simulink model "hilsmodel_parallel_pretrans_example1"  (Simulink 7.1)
settings: Solver=ode3  SolverMode=SingleTasking  StartTime=0.0  StopTime=1800  FixedStep=hilsmdl.simulation.stepsize.value  MaxStep=0.01  RelTol=1e-3  AbsTol=1e-3
undefined symbols (not defined in the file or in its folder): hilsmdl
libraries: HILS_model_library x10, simulink_extras x1, simulink x1

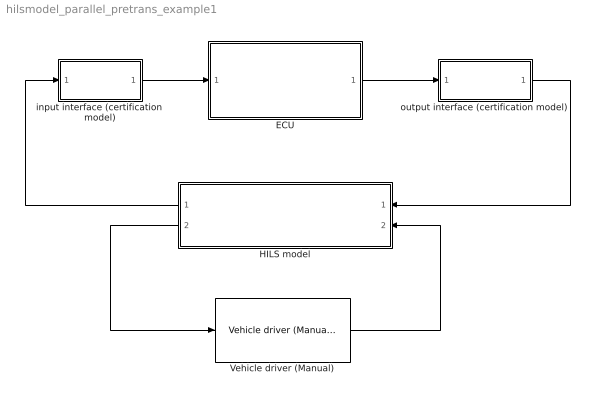
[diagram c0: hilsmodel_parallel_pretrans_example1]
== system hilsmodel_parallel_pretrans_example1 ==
  ECU : Subsystem  mask{dat=hilsmdl.ecu}
      mask prompts: dat "Data set for ECU"
  HILS model : Subsystem  Orientation=left
  Vehicle driver (Manual) : HILS_model_library/Driver/Vehicle driver (Manual)  dat=hilsmdl.drivermanual
  input interface (certification model) : Subsystem
  output interface (certification model) : Subsystem
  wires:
  input interface (certification model)/1(to ECU) -> ECU/1(sensor in)
  ECU/1(cmd out) -> output interface (certification model)/1(from ECU)
  HILS model/1(To Ctrl) -> input interface (certification model)/1(plant in)
  output interface (certification model)/1(cmd out) -> HILS model/1(From Ctrl)
  Vehicle driver (Manual)/1 -> HILS model/2(From Driver)
  HILS model/2(To driver) -> Vehicle driver (Manual)/1

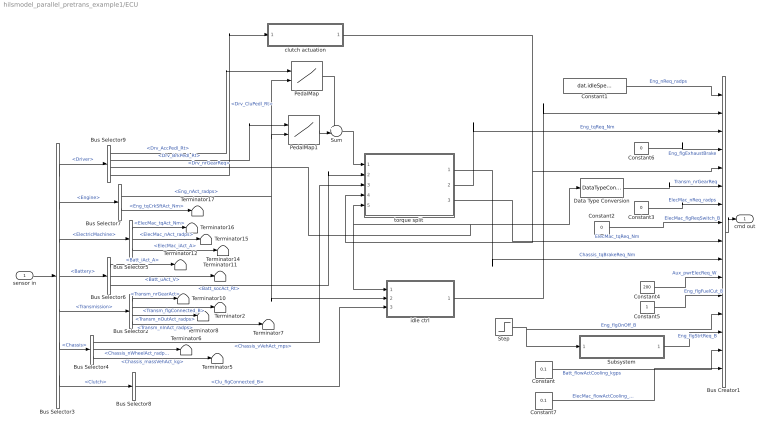
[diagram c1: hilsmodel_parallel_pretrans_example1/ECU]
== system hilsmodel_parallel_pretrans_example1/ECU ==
  sensor in : Inport
  Bus Creator1 : BusCreator  Inputs=16
  Bus Selector2 : BusSelector  OutputSignals=Transm_nrGearAct,Transm_flgConnected_B,Transm_nOutAct_radps,Transm_nInAct_radps
  Bus Selector3 : BusSelector  OutputSignals=Driver,Engine,ElectricMachine,Battery,Transmission,Chassis,Clutch
  Bus Selector4 : BusSelector  OutputSignals=Chassis_vVehAct_mps,Chassis_nWheelAct_radps,Chassis_massVehAct_kg
  Bus Selector5 : BusSelector  OutputSignals=ElecMac_tqAct_Nm,ElecMac_nAct_radps,ElecMac_iAct_A
  Bus Selector6 : BusSelector  OutputSignals=Batt_iAct_A,Batt_uAct_V,Batt_socAct_Rt
  Bus Selector7 : BusSelector  OutputSignals=Eng_nAct_radps,Eng_tqCrkSftAct_Nm
  Bus Selector8 : BusSelector  OutputSignals=Clu_flgConnected_B
  Bus Selector9 : BusSelector  OutputSignals=Drv_AccPedl_Rt,Drv_BrkPedl_Rt,Drv_nrGearReq,Drv_CluPedl_Rt
  Constant : Constant  Value=0.1
  Constant1 : Constant  Value=dat.idleSpeed.value
  Constant2 : Constant  Value=0
  Constant3 : Constant  Value=0
  Constant4 : Constant  Value=200
  Constant5 : Constant
  Constant6 : Constant  Value=0
  Constant7 : Constant  Value=0.1
  Data Type Conversion : DataTypeConversion
  PedalMap : Lookup2D  RowIndex=dat.pedalmap.pedal  ColumnIndex=dat.pedalmap.speed  Table=dat.pedalmap.map
  PedalMap1 : Lookup2D  RowIndex=dat.pedalmap.pedal  ColumnIndex=dat.pedalmap.speed  Table=2*dat.pedalmap.map
  Step : Step  SampleTime=0
  Subsystem : Subsystem
  Sum : Sum  Inputs=+-|
  Terminator{2,5..8,10..12,14..17} (12 alike) : Terminator
  clutch actuation : Subsystem
  idle ctrl : Subsystem
  torque split : Subsystem
  cmd out : Outport
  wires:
  Bus Selector3/6 -> Bus Selector4/1  "<Chassis>"
  Bus Selector3/5 -> Bus Selector2/1  "<Transmission>"
  Bus Selector3/3 -> Bus Selector5/1  "<ElectricMachine>"
  Bus Selector3/4 -> Bus Selector6/1  "<Battery>"
  sensor in/1 -> Bus Selector3/1
  Bus Creator1/1 -> cmd out/1
  Bus Selector6/1 -> Terminator12/1  "<Batt_iAct_A>"
  Bus Selector6/2 -> Terminator11/1  "<Batt_uAct_V>"
  Bus Selector6/3 -> torque split/2(SOC [0_1])  "<Batt_socAct_Rt>"
  Bus Selector2/1 -> Terminator10/1  "<Transm_nrGearAct>"
  Bus Selector2/2 -> Terminator2/1  "<Transm_flgConnected_B>"
  Bus Selector2/3 -> Terminator8/1  "<Transm_nOutAct_radps>"
  Bus Selector2/4 -> Terminator7/1  "<Transm_nInAct_radps>"
  Bus Selector5/3 -> Terminator14/1  "<ElecMac_iAct_A>"
  Bus Selector5/2 -> Terminator15/1  "<ElecMac_nAct_radps>"
  Bus Selector5/1 -> Terminator16/1  "<ElecMac_tqAct_Nm>"
  Bus Selector3/2 -> Bus Selector7/1  "<Engine>"
  Bus Selector7/2 -> Terminator17/1  "<Eng_tqCrkSftAct_Nm>"
  Bus Selector7/1 -> PedalMap/2, PedalMap1/2, idle ctrl/2(ICE_speed)  "<Eng_nAct_radps>"
  Bus Selector4/1 -> torque split/3(vehicle speed [m/s])  "<Chassis_vVehAct_mps>"
  Bus Selector4/2 -> Terminator6/1  "<Chassis_nWheelAct_radps>"
  Bus Selector4/3 -> Terminator5/1  "<Chassis_massVehAct_kg>"
  Bus Selector8/1 -> idle ctrl/3(CL_flag)  "<Clu_flgConnected_B>"
  PedalMap1/1 -> Sum/2
  PedalMap/1 -> Sum/1
  Sum/1 -> torque split/1(Tdemand [Nm])
  Bus Selector3/1 -> Bus Selector9/1  "<Driver>"
  Bus Selector9/1 -> PedalMap/1  "<Drv_AccPedl_Rt>"
  Bus Selector9/2 -> PedalMap1/1  "<Drv_BrkPedl_Rt>"
  Bus Selector3/7 -> Bus Selector8/1  "<Clutch>"
  Constant2/1 -> Bus Creator1/8  "ElecMac_flgReqSwitch_B"
  Constant3/1 -> Bus Creator1/7  "ElecMac_nReq_radps"
  Constant1/1 -> Bus Creator1/1  "Eng_nReq_radps"
  torque split/2(Treqice) -> Bus Creator1/3  "Eng_tqReq_Nm"
  torque split/3(Treqem) -> Bus Creator1/9  "ElecMac_tqReq_Nm"
  Constant6/1 -> Bus Creator1/4  "Eng_flgExhaustBrake"
  torque split/1(Tbrake) -> Bus Creator1/10  "Chassis_tqBrakeReq_Nm"
  Constant4/1 -> Bus Creator1/11  "Aux_pwrElecReq_W"
  Bus Selector9/3 -> Data Type Conversion/1, idle ctrl/1(gear), torque split/5(Gear [0_5])  "<Drv_nrGearReq>"
  Data Type Conversion/1 -> Bus Creator1/6  "Transm_nrGearReq"
  Bus Selector9/4 -> clutch actuation/1(In1)  "<Drv_CluPedl_Rt>"
  clutch actuation/1(Out1) -> torque split/4(Clutch [0;1]), Bus Creator1/5
  idle ctrl/1(Out1) -> Bus Creator1/2
  Constant5/1 -> Bus Creator1/12  "Eng_flgFuelCut_B"
  Step/1 -> Subsystem/1(Engine onoff), Bus Creator1/13  "Eng_flgOnOff_B"
  Subsystem/1(Starter motor ctrl) -> Bus Creator1/14  "Eng_flgStrtReq_B"
  Constant/1 -> Bus Creator1/15  "Batt_flowActCooling_kgps"
  Constant7/1 -> Bus Creator1/16  "ElecMac_flowActCooling_kgps"

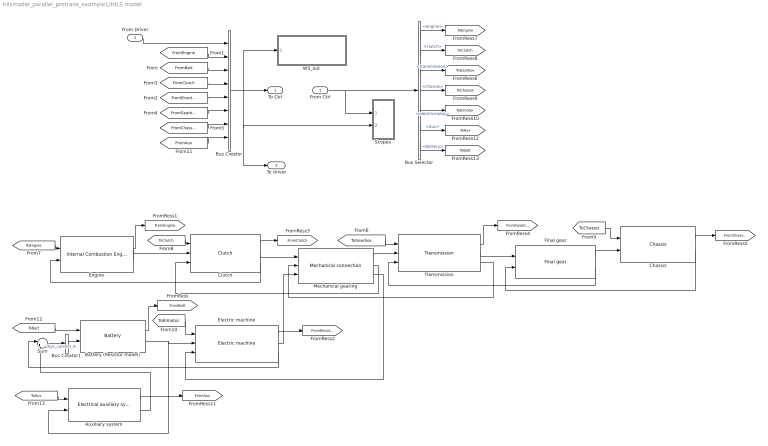
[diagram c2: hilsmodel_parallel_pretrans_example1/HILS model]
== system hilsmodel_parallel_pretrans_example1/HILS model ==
  From Ctrl : Inport
  From Driver : Inport  Port=2
  Auxiliary system : HILS_model_library/Auxiliary systems/Electrical auxiliary system
  Battery (Resistor model) : HILS_model_library/Rechargable energy storage systems/Battery  dat=hilsmdl.battery
  Bus Creator : BusCreator  Inputs=8
  Bus Creator1 : BusCreator  Inputs=1
  Bus Selector : BusSelector  OutputSignals=engine,clutch,transmission,chassis,electricmotor,aux,Battery
  Chassis : HILS_model_library/Chassis/Chassis  dat=hilsmdl.chassis
  Clutch : HILS_model_library/Mechanical components/Clutch  dat=hilsmdl.clutch
  Electric machine : HILS_model_library/Energy converters/Electric machine  dat=hilsmdl.elmachine
  Engine : HILS_model_library/Energy converters/Internal Combustion Engine  dat=hilsmdl.eng
  Final gear : HILS_model_library/Mechanical components/Final gear  dat=hilsmdl.finalgear
  Mechanical gearing : HILS_model_library/Mechanical components/Mechanical connection  dat=hilsmdl.mechconnection
  Scopes : Subsystem
  Sum : Sum  Inputs=|++
  Transmission : HILS_model_library/Mechanical components/Transmission  dat=hilsmdl.transmission
  WS_out : Subsystem
  To Ctrl : Outport
  To driver : Outport  Port=2
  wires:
  From Driver/1 -> Bus Creator/1
  Battery (Resistor model)/2 -> Electric machine/2, Auxiliary system/2
  Mechanical gearing/3 -> Electric machine/3
  Mechanical gearing/1 -> Transmission/2
  Bus Creator/1 -> To Ctrl/1, To driver/1, Scopes/2(plnt in), WS_out/1(from model)
  Clutch/2 -> Mechanical gearing/1
  Mechanical gearing/2 -> Clutch/3
  Clutch/3 -> Engine/2
  Transmission/3 -> Mechanical gearing/2
  Engine/2 -> Clutch/2
  Chassis/1 -> [FromChassis]
  From Ctrl/1 -> Scopes/1(ctrl in), Bus Selector/1
  Electric machine/2 -> Mechanical gearing/3
  Battery (Resistor model)/1 -> [FromBatt]
  [FromBatt] -> Bus Creator/3
  Engine/1 -> [FromEngine]
  [FromEngine] -> Bus Creator/2
  [FromElmotor] -> Bus Creator/5
  Electric machine/1 -> [FromElmotor]
  [FromClutch] -> Bus Creator/4
  Clutch/1 -> [FromClutch]
  [FromGearbox] -> Bus Creator/6
  Transmission/1 -> [FromGearbox]
  [FromChassis] -> Bus Creator/7
  Bus Selector/3 -> [ToGearbox]  "<transmission>"
  [ToGearbox] -> Transmission/1
  Bus Selector/1 -> [ToEngine]  "<engine>"
  Bus Selector/2 -> [ToClutch]  "<clutch>"
  Bus Selector/4 -> [ToChassis]  "<chassis>"
  Bus Selector/5 -> [ToElmotor]  "<electricmotor>"
  [ToEngine] -> Engine/1
  [ToClutch] -> Clutch/1
  [ToChassis] -> Chassis/1
  [ToElmotor] -> Electric machine/1
  [ToBatt] -> Battery (Resistor model)/1
  [ToAux] -> Auxiliary system/1
  Auxiliary system/1 -> [FromAux]
  [FromAux] -> Bus Creator/8
  Auxiliary system/2 -> Sum/2
  Electric machine/3 -> Sum/1
  Bus Creator1/1 -> Battery (Resistor model)/2
  Sum/1 -> Bus Creator1/1  "phys_current_A"
  Bus Selector/6 -> [ToAux]  "<aux>"
  Transmission/2 -> Final gear/1
  Final gear/2 -> Transmission/3
  Final gear/1 -> Chassis/2
  Chassis/2 -> Final gear/2
  Bus Selector/7 -> [ToBatt]  "<Battery>"

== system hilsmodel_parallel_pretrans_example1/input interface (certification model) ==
  plant in : Inport
  Bus Creator : BusCreator  Inputs=35
  Bus Selector : BusSelector  OutputSignals=Driver,Driver.Drv_AccPedl_Rt,Driver.Drv_BrkPedl_Rt,Driver.Drivecycle_RefSpeed_mps,Driver.Drv_CluPedl_Rt,Driver.Drv_nrGearReq,Engine,Engine.Eng_nAct_radps,Engine.Eng_tqCrkSftAct_Nm,Engine.Eng_tqIndAct_Nm,Engine.Eng_tOilAct_K,Battery,Battery.Batt_iAct_A,Battery.Batt_uAct_V,Battery.Batt_socAct_Rt,Battery.Batt_tAct_K,Clutch,Clutch.Clu_flgConnected_B,ElectricMachine,ElectricMachine.ElecMac_tqAct_Nm,Ele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
  to ECU : Outport
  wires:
  plant in/1 -> Bus Selector/1
  Bus Selector/1 -> Bus Creator/1  "<Driver>"
  Bus Selector/2 -> Bus Creator/2  "<Drv_AccPedl_Rt>"
  Bus Selector/3 -> Bus Creator/3  "<Drv_BrkPedl_Rt>"
  Bus Selector/4 -> Bus Creator/4  "<Drivecycle_RefSpeed_mps>"
  Bus Selector/5 -> Bus Creator/5  "<Drv_CluPedl_Rt>"
  Bus Selector/7 -> Bus Creator/7  "<Engine>"
  Bus Selector/8 -> Bus Creator/8  "<Eng_nAct_radps>"
  Bus Selector/9 -> Bus Creator/9  "<Eng_tqCrkSftAct_Nm>"
  Bus Selector/6 -> Bus Creator/6  "<Drv_nrGearReq>"
  Bus Creator/1 -> to ECU/1
  Bus Selector/10 -> Bus Creator/10  "<Eng_tqIndAct_Nm>"
  Bus Selector/11 -> Bus Creator/11  "<Eng_tOilAct_K>"
  Bus Selector/12 -> Bus Creator/12  "<Battery>"
  Bus Selector/13 -> Bus Creator/13  "<Batt_iAct_A>"
  Bus Selector/14 -> Bus Creator/14  "<Batt_uAct_V>"
  Bus Selector/15 -> Bus Creator/15  "<Batt_socAct_Rt>"
  Bus Selector/16 -> Bus Creator/16  "<Batt_tAct_K>"
  Bus Selector/17 -> Bus Creator/17  "<Clutch>"
  Bus Selector/18 -> Bus Creator/18  "<Clu_flgConnected_B>"
  Bus Selector/19 -> Bus Creator/19  "<ElectricMachine>"
  Bus Selector/20 -> Bus Creator/20  "<ElecMac_tqAct_Nm>"
  Bus Selector/21 -> Bus Creator/21  "<ElecMac_nAct_radps>"
  Bus Selector/22 -> Bus Creator/22  "<ElecMac_iAct_A>"
  Bus Selector/23 -> Bus Creator/23  "<ElecMac_tAct_K>"
  Bus Selector/24 -> Bus Creator/24  "<Transmission>"
  Bus Selector/25 -> Bus Creator/25  "<Transm_nOutAct_radps>"
  Bus Selector/26 -> Bus Creator/26  "<Transm_nrGearAct>"
  Bus Selector/27 -> Bus Creator/27  "<Transm_flgConnected_B>"
  Bus Selector/28 -> Bus Creator/28  "<Transm_nInAct_radps>"
  Bus Selector/29 -> Bus Creator/29  "<Chassis>"
  Bus Selector/30 -> Bus Creator/30  "<Chassis_vVehAct_mps>"
  Bus Selector/31 -> Bus Creator/31  "<Chassis_nWheelAct_radps>"
  Bus Selector/32 -> Bus Creator/32  "<Chassis_massVehAct_kg>"
  Bus Selector/33 -> Bus Creator/33  "<Chassis_slopRoad_rad>"
  Bus Selector/34 -> Bus Creator/34  "<Auxiliary>"
  Bus Selector/35 -> Bus Creator/35  "<Aux_iAct_A>"

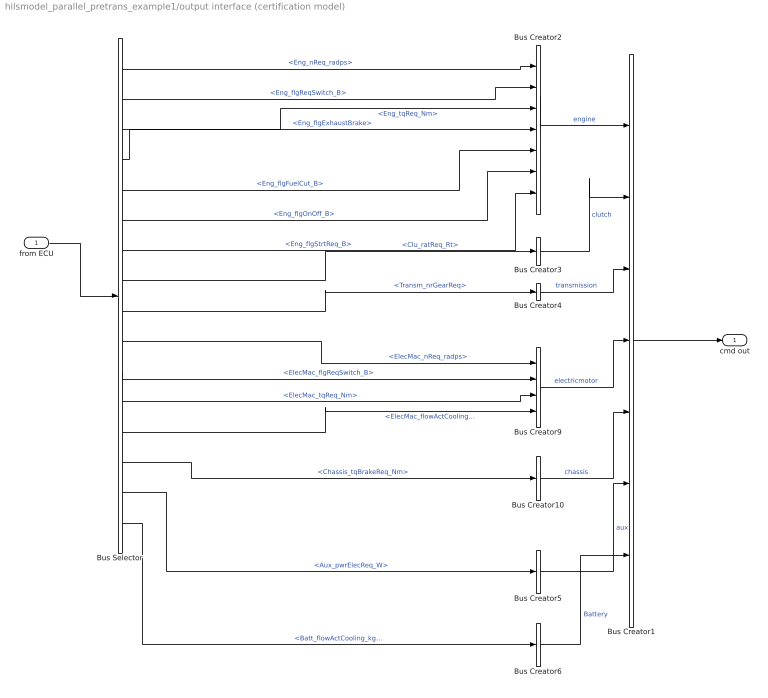
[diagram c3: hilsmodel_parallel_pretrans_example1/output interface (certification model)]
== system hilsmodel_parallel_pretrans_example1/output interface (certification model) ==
  from ECU : Inport
  Bus Creator1 : BusCreator  Inputs=7
  Bus Creator{3..6,10} (5 alike) : BusCreator  Inputs=1
  Bus Creator2 : BusCreator  Inputs=7
  Bus Creator9 : BusCreator
  Bus Selector : BusSelector  OutputSignals=Eng_nReq_radps,Eng_flgReqSwitch_B,Eng_tqReq_Nm,Eng_flgExhaustBrake,Eng_flgFuelCut_B,Eng_flgOnOff_B,Eng_flgStrtReq_B,Clu_ratReq_Rt,Transm_nrGearReq,ElecMac_nReq_radps,ElecMac_flgReqSwitch_B,ElecMac_tqReq_Nm,ElecMac_flowActCooling_kgps,Chassis_tqBrakeReq_Nm,Aux_pwrElecReq_W,Batt_flowActCooling_kgps
  cmd out : Outport
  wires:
  from ECU/1 -> Bus Selector/1
  Bus Creator4/1 -> Bus Creator1/3  "transmission"
  Bus Creator3/1 -> Bus Creator1/2  "clutch"
  Bus Creator10/1 -> Bus Creator1/5  "chassis"
  Bus Creator9/1 -> Bus Creator1/4  "electricmotor"
  Bus Selector/11 -> Bus Creator9/2  "<ElecMac_flgReqSwitch_B>"
  Bus Selector/10 -> Bus Creator9/1  "<ElecMac_nReq_radps>"
  Bus Creator1/1 -> cmd out/1
  Bus Creator2/1 -> Bus Creator1/1  "engine"
  Bus Selector/1 -> Bus Creator2/1  "<Eng_nReq_radps>"
  Bus Selector/2 -> Bus Creator2/2  "<Eng_flgReqSwitch_B>"
  Bus Selector/3 -> Bus Creator2/3  "<Eng_tqReq_Nm>"
  Bus Selector/12 -> Bus Creator9/3  "<ElecMac_tqReq_Nm>"
  Bus Selector/4 -> Bus Creator2/4  "<Eng_flgExhaustBrake>"
  Bus Selector/8 -> Bus Creator3/1  "<Clu_ratReq_Rt>"
  Bus Selector/9 -> Bus Creator4/1  "<Transm_nrGearReq>"
  Bus Selector/14 -> Bus Creator10/1  "<Chassis_tqBrakeReq_Nm>"
  Bus Creator5/1 -> Bus Creator1/6  "aux"
  Bus Selector/15 -> Bus Creator5/1  "<Aux_pwrElecReq_W>"
  Bus Selector/5 -> Bus Creator2/5  "<Eng_flgFuelCut_B>"
  Bus Selector/6 -> Bus Creator2/6  "<Eng_flgOnOff_B>"
  Bus Selector/7 -> Bus Creator2/7  "<Eng_flgStrtReq_B>"
  Bus Selector/16 -> Bus Creator6/1  "<Batt_flowActCooling_kgps>"
  Bus Creator6/1 -> Bus Creator1/7  "Battery"
  Bus Selector/13 -> Bus Creator9/4  "<ElecMac_flowActCooling_kgps>"

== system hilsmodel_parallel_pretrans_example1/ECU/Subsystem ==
  Engine onoff : Inport
  Data Type Conversion : DataTypeConversion
  Data Type Conversion1 : DataTypeConversion
  S-R Flip-Flop : simulink_extras/Flip Flops/S-R Flip-Flop  initial_condition=0
  Terminator : Terminator
  Transport Delay : TransportDelay
  Starter motor ctrl : Outport
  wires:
  Engine onoff/1 -> Transport Delay/1, Data Type Conversion/1
  S-R Flip-Flop/1 -> Starter motor ctrl/1
  S-R Flip-Flop/2 -> Terminator/1
  Transport Delay/1 -> Data Type Conversion1/1
  Data Type Conversion/1 -> S-R Flip-Flop/1
  Data Type Conversion1/1 -> S-R Flip-Flop/2

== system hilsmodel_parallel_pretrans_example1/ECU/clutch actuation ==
  In1 : Inport
  Gain : Gain
  Scope : Scope
  Out1 : Outport
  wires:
  In1/1 -> Gain/1
  Gain/1 -> Out1/1, Scope/1  "Clu_ratReq_Rt"

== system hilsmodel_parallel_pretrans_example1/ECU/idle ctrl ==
  gear : Inport
  ICE_speed : Inport  Port=2
  CL_flag : Inport  Port=3
  Compare To Zero : simulink/Logic and Bit Operations/Compare To Zero  relop=<=  LogicOutDataTypeMode=boolean
  Const2 : Constant  Value=dat.idleSpeed.value
  Logical Operator : Logic  Operator=NOT  AllPortsSameDT=off  OutDataTypeStr=boolean  OutDataTypeMode=boolean
  Logical Operator1 : Logic  Operator=OR  AllPortsSameDT=off  OutDataTypeStr=boolean  OutDataTypeMode=boolean
  Logical Operator2 : Logic  Operator=OR  AllPortsSameDT=off  OutDataTypeStr=boolean  OutDataTypeMode=boolean
  Relational Operator1 : RelationalOperator  Operator=<  OutDataTypeStr=boolean  LogicOutDataTypeMode=boolean
  Out1 : Outport
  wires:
  Compare To Zero/1 -> Logical Operator1/1
  Relational Operator1/1 -> Logical Operator2/1
  Const2/1 -> Relational Operator1/2
  gear/1 -> Compare To Zero/1
  ICE_speed/1 -> Relational Operator1/1
  Logical Operator1/1 -> Out1/1  "Eng_flgReqSwitch_B"
  Logical Operator2/1 -> Logical Operator1/2
  CL_flag/1 -> Logical Operator/1
  Logical Operator/1 -> Logical Operator2/2

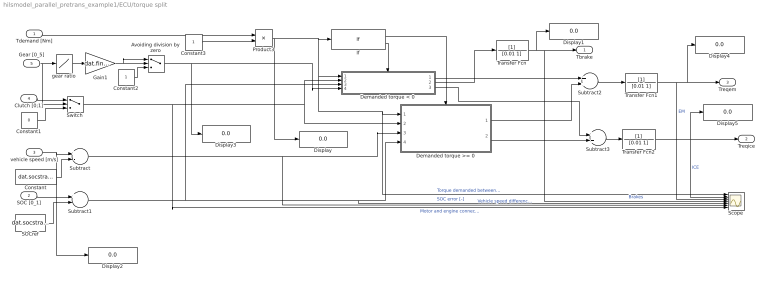
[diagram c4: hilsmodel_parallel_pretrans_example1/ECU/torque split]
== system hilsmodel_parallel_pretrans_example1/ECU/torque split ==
  Tdemand [Nm] : Inport
  SOC [0_1] : Inport  Port=2
  vehicle speed [m/s] : Inport  Port=3
  Clutch [0;1] : Inport  Port=4
  Gear [0_5] : Inport  Port=5
  Avoiding division by zero : Switch  Criteria=u2 > Threshold  Threshold=0.1
  Constant : Constant  Value=dat.socstrategy.SwitchSpeed
  Constant1 : Constant  Value=0
  Constant2 : Constant
  Constant3 : Constant
  Demanded torque < 0 : Subsystem  TreatAsAtomicUnit=on
  Demanded torque >= 0 : Subsystem  TreatAsAtomicUnit=on
  Display{,1..5} (6 alike) : Display
  Gain1 : Gain  Gain=dat.finalgear.value
  If : If  IfExpression=u1 >=0
  Product3 : Product  Inputs=*/
  SOCref : Constant  Value=dat.socstrategy.socref
  Scope : Scope  NumInputPorts=7
  Subtract : Sum  Inputs=+-
  Subtract1 : Sum  Inputs=+-
  Subtract2 : Sum
  Subtract3 : Sum
  Switch : Switch  Threshold=0.5
  Transfer Fcn : TransferFcn  Denominator=[0.01 1]
  Transfer Fcn1 : TransferFcn  Denominator=[0.01 1]
  Transfer Fcn2 : TransferFcn  Denominator=[0.01 1]
  gear ratio : Lookup  InputValues=dat.gearname.value  Table=dat.gearratio.value
  Tbrake : Outport
  Treqice : Outport  Port=2
  Treqem : Outport  Port=3
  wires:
  Gear [0_5]/1 -> gear ratio/1, Switch/2
  Tdemand [Nm]/1 -> Product3/1
  gear ratio/1 -> Gain1/1
  Product3/1 -> If/1, Demanded torque < 0/1(Tdemand [Nm]), Demanded torque >= 0/1(Tdemand [Nm]), Scope/1, Display/1  "Torque demanded between clutch and EM/ICE"
  Clutch [0;1]/1 -> Switch/1
  Constant1/1 -> Switch/3
  Switch/1 -> Demanded torque < 0/2(Connected? [0;1]), Demanded torque >= 0/2(Connected? [0;1]), Scope/7  "Motor and engine connected to wheels ?"
  vehicle speed [m/s]/1 -> Subtract/1, Display2/1
  Constant/1 -> Subtract/2
  Subtract/1 -> Demanded torque >= 0/3(Switch diff [m/s]), Scope/6  "Vehicle speed difference from  EM/ICE switch speed [m/s]"
  SOC [0_1]/1 -> Subtract1/1
  SOCref/1 -> Subtract1/2
  Subtract1/1 -> Demanded torque < 0/3(SOC error), Demanded torque >= 0/4(SOC error [-]), Scope/5  "SOC error [-]"
  If/1 -> Demanded torque >= 0/Action
  If/2 -> Demanded torque < 0/Action
  Demanded torque < 0/1(Torque EM) -> Subtract2/1
  Demanded torque >= 0/1(Torque EM) -> Subtract2/2
  Subtract2/1 -> Transfer Fcn1/1
  Demanded torque < 0/2(Torque brakes) -> Transfer Fcn/1
  Gain1/1 -> Avoiding division by zero/2, Avoiding division by zero/1
  Constant2/1 -> Avoiding division by zero/3
  Avoiding division by zero/1 -> Demanded torque < 0/4(Gear ratio), Display3/1
  Demanded torque >= 0/2(Torque ICE) -> Subtract3/2
  Demanded torque < 0/3(Torque ICE) -> Subtract3/1
  Subtract3/1 -> Transfer Fcn2/1
  Transfer Fcn/1 -> Display1/1, Tbrake/1, Scope/4  "Brakes"
  Transfer Fcn1/1 -> Treqem/1, Display4/1, Scope/3  "EM"
  Transfer Fcn2/1 -> Treqice/1, Display5/1, Scope/2  "ICE"
  Constant3/1 -> Product3/2

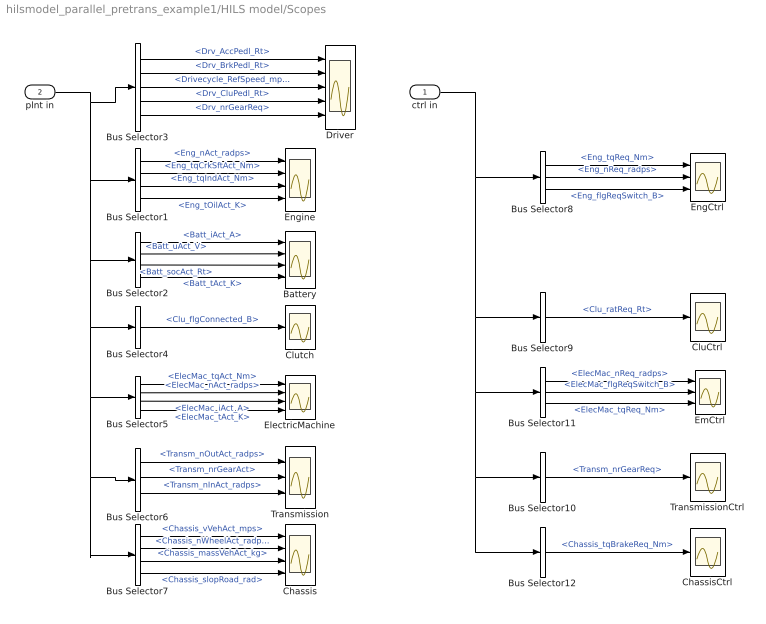
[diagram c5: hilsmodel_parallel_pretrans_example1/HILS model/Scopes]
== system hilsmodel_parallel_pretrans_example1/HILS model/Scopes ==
  ctrl in : Inport
  plnt in : Inport  Port=2
  Battery : Scope  NumInputPorts=4
  Bus Selector1 : BusSelector  OutputSignals=Engine.Eng_nAct_radps,Engine.Eng_tqCrkSftAct_Nm,Engine.Eng_tqIndAct_Nm,Engine.Eng_tOilAct_K
  Bus Selector10 : BusSelector  OutputSignals=transmission.Transm_nrGearReq
  Bus Selector11 : BusSelector  OutputSignals=electricmotor.ElecMac_nReq_radps,electricmotor.ElecMac_flgReqSwitch_B,electricmotor.ElecMac_tqReq_Nm
  Bus Selector12 : BusSelector  OutputSignals=chassis.Chassis_tqBrakeReq_Nm
  Bus Selector2 : BusSelector  OutputSignals=Battery.Batt_iAct_A,Battery.Batt_uAct_V,Battery.Batt_socAct_Rt,Battery.Batt_tAct_K
  Bus Selector3 : BusSelector  OutputSignals=Driver.Drv_AccPedl_Rt,Driver.Drv_BrkPedl_Rt,Driver.Drivecycle_RefSpeed_mps,Driver.Drv_CluPedl_Rt,Driver.Drv_nrGearReq
  Bus Selector4 : BusSelector  OutputSignals=Clutch.Clu_flgConnected_B
  Bus Selector5 : BusSelector  OutputSignals=ElectricMachine.ElecMac_tqAct_Nm,ElectricMachine.ElecMac_nAct_radps,ElectricMachine.ElecMac_iAct_A,ElectricMachine.ElecMac_tAct_K
  Bus Selector6 : BusSelector  OutputSignals=Transmission.Transm_nOutAct_radps,Transmission.Transm_nrGearAct,Transmission.Transm_nInAct_radps,Transmission.Transm_flgConnected_B
  Bus Selector7 : BusSelector  OutputSignals=Chassis.Chassis_vVehAct_mps,Chassis.Chassis_nWheelAct_radps,Chassis.Chassis_massVehAct_kg,Chassis.Chassis_slopRoad_rad
  Bus Selector8 : BusSelector  OutputSignals=engine.Eng_tqReq_Nm,engine.Eng_nReq_radps,engine.Eng_flgReqSwitch_B
  Bus Selector9 : BusSelector  OutputSignals=clutch.Clu_ratReq_Rt
  Chassis : Scope  NumInputPorts=4
  ChassisCtrl : Scope
  CluCtrl : Scope
  Clutch : Scope
  Driver : Scope  NumInputPorts=5
  ElectricMachine : Scope  NumInputPorts=4
  EmCtrl : Scope  NumInputPorts=3
  EngCtrl : Scope  NumInputPorts=3
  Engine : Scope  NumInputPorts=4
  Transmission : Scope  NumInputPorts=3
  TransmissionCtrl : Scope
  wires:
  Bus Selector3/1 -> Driver/1  "<Drv_AccPedl_Rt>"
  Bus Selector3/3 -> Driver/3  "<Drivecycle_RefSpeed_mps>"
  Bus Selector3/2 -> Driver/2  "<Drv_BrkPedl_Rt>"
  plnt in/1 -> Bus Selector3/1, Bus Selector1/1, Bus Selector2/1, Bus Selector4/1, Bus Selector5/1, Bus Selector6/1, Bus Selector7/1
  Bus Selector1/1 -> Engine/1  "<Eng_nAct_radps>"
  Bus Selector1/2 -> Engine/2  "<Eng_tqCrkSftAct_Nm>"
  Bus Selector2/1 -> Battery/1  "<Batt_iAct_A>"
  Bus Selector2/2 -> Battery/2  "<Batt_uAct_V>"
  Bus Selector2/3 -> Battery/3  "<Batt_socAct_Rt>"
  Bus Selector4/1 -> Clutch/1  "<Clu_flgConnected_B>"
  Bus Selector5/1 -> ElectricMachine/1  "<ElecMac_tqAct_Nm>"
  Bus Selector5/2 -> ElectricMachine/2  "<ElecMac_nAct_radps>"
  Bus Selector6/1 -> Transmission/1  "<Transm_nOutAct_radps>"
  Bus Selector6/2 -> Transmission/2  "<Transm_nrGearAct>"
  Bus Selector6/3 -> Transmission/3  "<Transm_nInAct_radps>"
  Bus Selector7/1 -> Chassis/1  "<Chassis_vVehAct_mps>"
  Bus Selector7/2 -> Chassis/2  "<Chassis_nWheelAct_radps>"
  Bus Selector7/3 -> Chassis/3  "<Chassis_massVehAct_kg>"
  Bus Selector7/4 -> Chassis/4  "<Chassis_slopRoad_rad>"
  ctrl in/1 -> Bus Selector8/1, Bus Selector9/1, Bus Selector11/1, Bus Selector10/1, Bus Selector12/1
  Bus Selector8/1 -> EngCtrl/1  "<Eng_tqReq_Nm>"
  Bus Selector8/2 -> EngCtrl/2  "<Eng_nReq_radps>"
  Bus Selector9/1 -> CluCtrl/1  "<Clu_ratReq_Rt>"
  Bus Selector10/1 -> TransmissionCtrl/1  "<Transm_nrGearReq>"
  Bus Selector11/1 -> EmCtrl/1  "<ElecMac_nReq_radps>"
  Bus Selector11/2 -> EmCtrl/2  "<ElecMac_flgReqSwitch_B>"
  Bus Selector11/3 -> EmCtrl/3  "<ElecMac_tqReq_Nm>"
  Bus Selector12/1 -> ChassisCtrl/1  "<Chassis_tqBrakeReq_Nm>"
  Bus Selector8/3 -> EngCtrl/3  "<Eng_flgReqSwitch_B>"
  Bus Selector1/3 -> Engine/3  "<Eng_tqIndAct_Nm>"
  Bus Selector1/4 -> Engine/4  "<Eng_tOilAct_K>"
  Bus Selector2/4 -> Battery/4  "<Batt_tAct_K>"
  Bus Selector5/3 -> ElectricMachine/3  "<ElecMac_iAct_A>"
  Bus Selector5/4 -> ElectricMachine/4  "<ElecMac_tAct_K>"
  Bus Selector3/4 -> Driver/4  "<Drv_CluPedl_Rt>"
  Bus Selector3/5 -> Driver/5  "<Drv_nrGearReq>"

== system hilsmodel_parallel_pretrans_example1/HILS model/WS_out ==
  from model : Inport
  To Workspace : ToWorkspace  VariableName=certmdl_out  SampleTime=hilsmdl.simulation.sampletime.value  SaveFormat=Structure With Time
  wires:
  from model/1 -> To Workspace/1

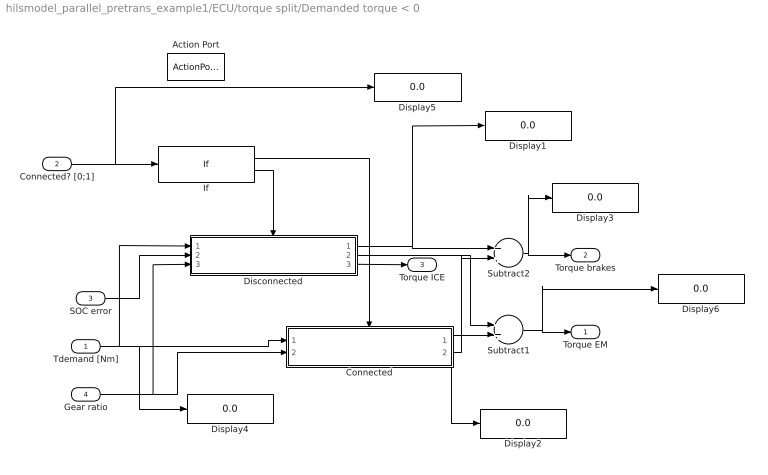
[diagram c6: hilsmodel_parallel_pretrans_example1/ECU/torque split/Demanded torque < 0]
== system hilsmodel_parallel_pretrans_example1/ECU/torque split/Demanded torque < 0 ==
  Tdemand [Nm] : Inport
  Connected? [0;1] : Inport  Port=2
  SOC error : Inport  Port=3
  Gear ratio : Inport  Port=4
  Action Port : ActionPort  InitializeStates=reset  ActionType=else
  Connected : Subsystem  TreatAsAtomicUnit=on
  Disconnected : Subsystem  TreatAsAtomicUnit=on
  Display{1..6} (6 alike) : Display
  If : If  IfExpression=u1 > 0.5
  Subtract1 : Sum
  Subtract2 : Sum
  Torque EM : Outport  OutputWhenDisabled=reset  InitialOutput=[0]
  Torque brakes : Outport  Port=2  OutputWhenDisabled=reset  InitialOutput=[0]
  Torque ICE : Outport  Port=3
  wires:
  If/1 -> Connected/Action
  If/2 -> Disconnected/Action
  Disconnected/1(Torque brakes) -> Subtract2/1, Display1/1
  Connected/2(Torque brakes) -> Subtract2/2, Display2/1
  Subtract2/1 -> Torque brakes/1, Display3/1
  Tdemand [Nm]/1 -> Disconnected/1(Tdemand [Nm]), Connected/1(Tdemand [Nm]), Display4/1
  Connected/1(Torque EM) -> Subtract1/2
  Disconnected/2(Torque EM) -> Subtract1/1
  Subtract1/1 -> Torque EM/1, Display6/1
  Disconnected/3(Torque ICE) -> Torque ICE/1
  SOC error/1 -> Disconnected/2(SOC error)
  Connected? [0;1]/1 -> If/1, Display5/1
  Gear ratio/1 -> Connected/2(Gear ratio), Disconnected/3(Gear ratio)

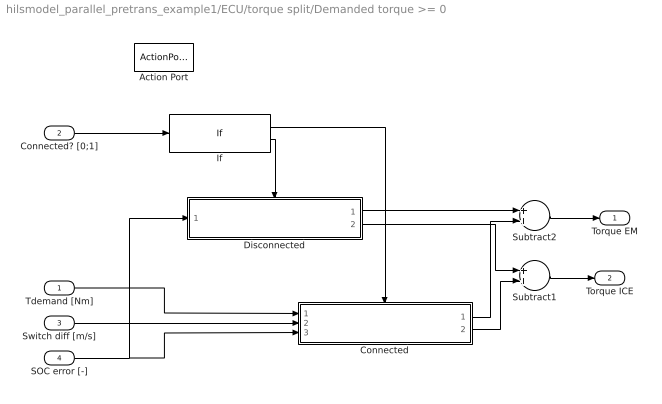
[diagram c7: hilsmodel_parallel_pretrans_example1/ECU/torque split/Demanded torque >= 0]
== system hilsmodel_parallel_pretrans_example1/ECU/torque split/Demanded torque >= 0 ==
  Tdemand [Nm] : Inport
  Connected? [0;1] : Inport  Port=2
  Switch diff [m/s] : Inport  Port=3
  SOC error [-] : Inport  Port=4
  Action Port : ActionPort  InitializeStates=reset  ActionType=then
  Connected : Subsystem  TreatAsAtomicUnit=on
  Disconnected : Subsystem  TreatAsAtomicUnit=on
  If : If  IfExpression=u1 > 0.5
  Subtract1 : Sum
  Subtract2 : Sum
  Torque EM : Outport  OutputWhenDisabled=reset  InitialOutput=[0]
  Torque ICE : Outport  Port=2  OutputWhenDisabled=reset  InitialOutput=[0]
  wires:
  If/1 -> Connected/Action
  If/2 -> Disconnected/Action
  Connected? [0;1]/1 -> If/1
  Switch diff [m/s]/1 -> Connected/2(Switch diff [m/s])
  SOC error [-]/1 -> Connected/3(SOC error), Disconnected/1(SOC error)
  Connected/1(Torque EM) -> Subtract2/2
  Tdemand [Nm]/1 -> Connected/1(Tdemand [Nm])
  Disconnected/1(Torque EM) -> Subtract2/1
  Connected/2(Torque ICE) -> Subtract1/2
  Disconnected/2(Torque ICE) -> Subtract1/1
  Subtract2/1 -> Torque EM/1
  Subtract1/1 -> Torque ICE/1

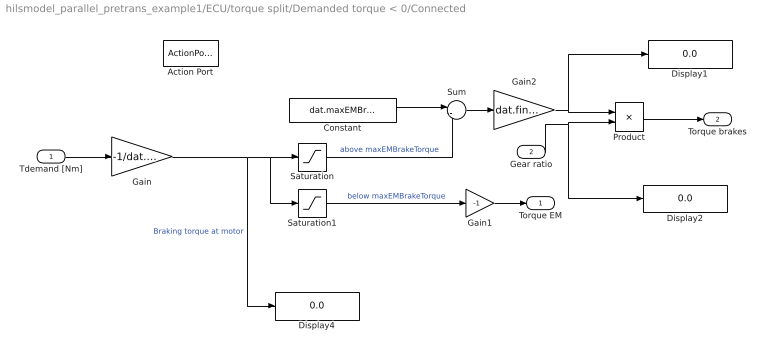
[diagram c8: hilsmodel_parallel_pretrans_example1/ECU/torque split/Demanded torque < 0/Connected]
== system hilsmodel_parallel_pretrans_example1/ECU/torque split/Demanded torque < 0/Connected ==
  Tdemand [Nm] : Inport
  Gear ratio : Inport  Port=2
  Action Port : ActionPort  InitializeStates=reset  ActionType=then
  Constant : Constant  Value=dat.maxEMBrakeTorque.value
  Display1 : Display
  Display2 : Display
  Display4 : Display
  Gain : Gain  Gain=-1/dat.finalgear.value
  Gain1 : Gain  Gain=-1
  Gain2 : Gain  Gain=dat.finalgear.value
  Product : Product
  Saturation : Saturate  UpperLimit=inf  LowerLimit=dat.maxEMBrakeTorque.value
  Saturation1 : Saturate  UpperLimit=dat.maxEMBrakeTorque.value  LowerLimit=-inf
  Sum : Sum  Inputs=|-+
  Torque EM : Outport  OutputWhenDisabled=reset  InitialOutput=[0]
  Torque brakes : Outport  Port=2  OutputWhenDisabled=reset  InitialOutput=[0]
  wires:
  Tdemand [Nm]/1 -> Gain/1
  Gain/1 -> Saturation/1, Saturation1/1, Display4/1  "Braking torque at motor"
  Saturation1/1 -> Gain1/1  "below maxEMBrakeTorque"
  Saturation/1 -> Sum/2  "above maxEMBrakeTorque"
  Constant/1 -> Sum/1
  Sum/1 -> Gain2/1
  Gain1/1 -> Torque EM/1
  Gain2/1 -> Display1/1, Product/1
  Product/1 -> Torque brakes/1
  Gear ratio/1 -> Product/2, Display2/1

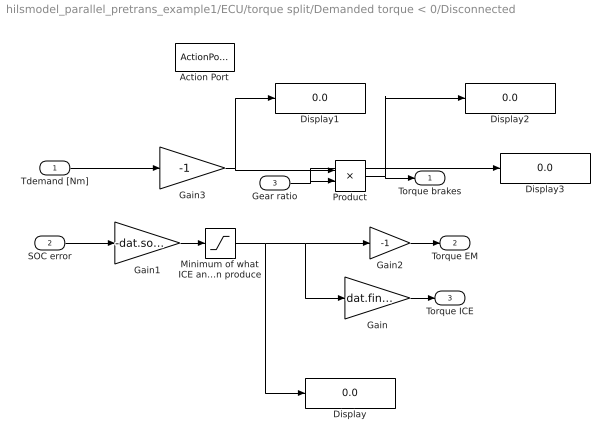
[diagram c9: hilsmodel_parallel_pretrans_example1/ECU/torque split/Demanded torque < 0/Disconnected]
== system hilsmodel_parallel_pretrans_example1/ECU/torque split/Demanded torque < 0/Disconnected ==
  Tdemand [Nm] : Inport
  SOC error : Inport  Port=2
  Gear ratio : Inport  Port=3
  Action Port : ActionPort  InitializeStates=reset  ActionType=else
  Display{,1..3} (4 alike) : Display
  Gain : Gain  Gain=dat.finalgear.value
  Gain1 : Gain  Gain=-dat.socstrategy.Ksoc
  Gain2 : Gain  Gain=-1
  Gain3 : Gain  Gain=-1
  Minimum of what ICE and EM can produce : Saturate  UpperLimit=min(dat.maxEMTorque.value,dat.maxEngineTorque.value/dat.finalgear.value)  LowerLimit=0
  Product : Product
  Torque brakes : Outport  OutputWhenDisabled=reset  InitialOutput=[0]
  Torque EM : Outport  Port=2  OutputWhenDisabled=reset  InitialOutput=[0]
  Torque ICE : Outport  Port=3  OutputWhenDisabled=reset  InitialOutput=[0]
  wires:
  Tdemand [Nm]/1 -> Gain3/1
  Gain1/1 -> Minimum of what ICE and EM can produce/1
  Minimum of what ICE and EM can produce/1 -> Gain2/1, Gain/1, Display/1
  SOC error/1 -> Gain1/1
  Gain2/1 -> Torque EM/1
  Gain/1 -> Torque ICE/1
  Gain3/1 -> Product/1, Display1/1
  Gear ratio/1 -> Product/2, Display3/1
  Product/1 -> Torque brakes/1, Display2/1

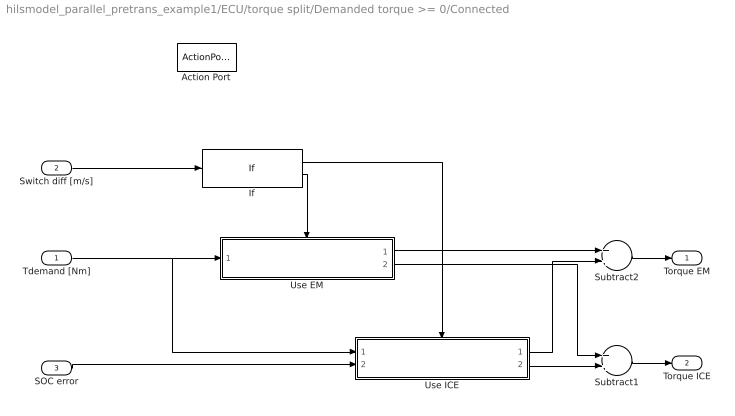
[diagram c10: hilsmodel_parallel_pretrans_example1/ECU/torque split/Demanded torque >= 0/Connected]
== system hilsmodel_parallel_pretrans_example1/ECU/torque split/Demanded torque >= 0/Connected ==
  Tdemand [Nm] : Inport
  Switch diff [m/s] : Inport  Port=2
  SOC error : Inport  Port=3
  Action Port : ActionPort  InitializeStates=reset  ActionType=then
  If : If
  Subtract1 : Sum
  Subtract2 : Sum
  Use EM : Subsystem  TreatAsAtomicUnit=on
  Use ICE : Subsystem  TreatAsAtomicUnit=on
  Torque EM : Outport  OutputWhenDisabled=reset  InitialOutput=[0]
  Torque ICE : Outport  Port=2  OutputWhenDisabled=reset  InitialOutput=[0]
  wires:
  If/1 -> Use ICE/Action
  If/2 -> Use EM/Action
  Tdemand [Nm]/1 -> Use ICE/1(Tdemand [Nm]), Use EM/1(Tdemand [Nm])
  Switch diff [m/s]/1 -> If/1
  SOC error/1 -> Use ICE/2(SOC error)
  Use EM/1(Torque EM) -> Subtract2/1
  Use ICE/1(Torque EM) -> Subtract2/2
  Use EM/2(Torque ICE) -> Subtract1/1
  Use ICE/2(Torque ICE) -> Subtract1/2
  Subtract1/1 -> Torque ICE/1
  Subtract2/1 -> Torque EM/1

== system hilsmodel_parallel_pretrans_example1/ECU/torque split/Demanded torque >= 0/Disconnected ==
  SOC error : Inport
  Action Port : ActionPort  InitializeStates=reset  ActionType=else
  Display : Display
  Gain : Gain  Gain=dat.finalgear.value
  Gain1 : Gain  Gain=-dat.socstrategy.Ksoc
  Gain2 : Gain  Gain=-1
  Minimum of what ICE and EM can produce : Saturate  UpperLimit=min(dat.maxEMTorque.value,dat.maxEngineTorque.value/dat.finalgear.value)  LowerLimit=0
  Torque EM : Outport  OutputWhenDisabled=reset  InitialOutput=[0]
  Torque ICE : Outport  Port=2  OutputWhenDisabled=reset  InitialOutput=[0]
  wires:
  Gain1/1 -> Minimum of what ICE and EM can produce/1
  Minimum of what ICE and EM can produce/1 -> Gain2/1, Gain/1, Display/1
  SOC error/1 -> Gain1/1
  Gain2/1 -> Torque EM/1
  Gain/1 -> Torque ICE/1

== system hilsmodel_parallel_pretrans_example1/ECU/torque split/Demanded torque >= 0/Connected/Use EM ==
  Tdemand [Nm] : Inport
  Action Port : ActionPort  InitializeStates=reset  ActionType=else
  Constant : Constant  Value=dat.maxEMTorque.value
  Gain : Gain  Gain=1/dat.finalgear.value
  Gain2 : Gain  Gain=dat.finalgear.value
  Saturation : Saturate  UpperLimit=inf  LowerLimit=dat.maxEMTorque.value
  Saturation1 : Saturate  UpperLimit=dat.maxEMTorque.value  LowerLimit=-inf
  Sum : Sum  Inputs=|-+
  Torque EM : Outport  OutputWhenDisabled=reset  InitialOutput=[0]
  Torque ICE : Outport  Port=2  OutputWhenDisabled=reset  InitialOutput=[0]
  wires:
  Tdemand [Nm]/1 -> Gain/1
  Gain/1 -> Saturation/1, Saturation1/1  "torque ref  at motor"
  Saturation1/1 -> Torque EM/1
  Saturation/1 -> Sum/2
  Constant/1 -> Sum/1
  Sum/1 -> Gain2/1
  Gain2/1 -> Torque ICE/1

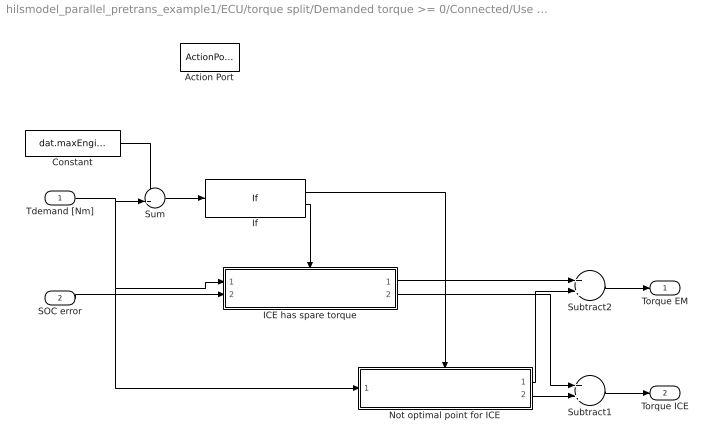
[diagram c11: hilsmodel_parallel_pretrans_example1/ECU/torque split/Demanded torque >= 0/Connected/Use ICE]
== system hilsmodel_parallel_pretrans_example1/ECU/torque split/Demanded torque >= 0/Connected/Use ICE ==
  Tdemand [Nm] : Inport
  SOC error : Inport  Port=2
  Action Port : ActionPort  InitializeStates=reset  ActionType=then
  Constant : Constant  Value=dat.maxEngineTorque.value
  ICE has spare torque : Subsystem  TreatAsAtomicUnit=on
  If : If
  Not optimal point for ICE : Subsystem  TreatAsAtomicUnit=on
  Subtract1 : Sum
  Subtract2 : Sum
  Sum : Sum  Inputs=-+|
  Torque EM : Outport  OutputWhenDisabled=reset  InitialOutput=[0]
  Torque ICE : Outport  Port=2  OutputWhenDisabled=reset  InitialOutput=[0]
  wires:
  If/1 -> Not optimal point for ICE/Action
  If/2 -> ICE has spare torque/Action
  Tdemand [Nm]/1 -> Sum/2, Not optimal point for ICE/1(Tdemand [Nm]), ICE has spare torque/1(Tdemand [Nm])
  Constant/1 -> Sum/1
  Sum/1 -> If/1
  Not optimal point for ICE/1(Torque EM) -> Subtract2/2
  Subtract2/1 -> Torque EM/1
  Not optimal point for ICE/2(Torque ICE) -> Subtract1/2
  Subtract1/1 -> Torque ICE/1
  SOC error/1 -> ICE has spare torque/2(SOC error)
  ICE has spare torque/2(Torque ICE) -> Subtract1/1
  ICE has spare torque/1(Torque EM) -> Subtract2/1

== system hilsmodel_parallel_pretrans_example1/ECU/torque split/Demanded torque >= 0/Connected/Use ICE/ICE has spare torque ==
  Tdemand [Nm] : Inport
  SOC error : Inport  Port=2
  Action Port : ActionPort  InitializeStates=reset  ActionType=else
  Gain : Gain  Gain=-1/dat.finalgear.value
  Gain1 : Gain  Gain=-dat.socstrategy.Ksoc
  Saturation : Saturate  UpperLimit=inf  LowerLimit=0
  Saturation2 : Saturate  UpperLimit=dat.maxEngineTorque.value  LowerLimit=0
  Sum1 : Sum  Inputs=|++
  Sum2 : Sum  Inputs=|-+
  Torque EM : Outport  OutputWhenDisabled=reset  InitialOutput=[0]
  Torque ICE : Outport  Port=2  OutputWhenDisabled=reset  InitialOutput=[0]
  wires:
  SOC error/1 -> Gain1/1
  Gain1/1 -> Saturation/1
  Saturation/1 -> Sum1/2  "Torque for charging >0 if SOC<SOC ref"
  Tdemand [Nm]/1 -> Sum1/1, Sum2/1
  Sum1/1 -> Saturation2/1
  Saturation2/1 -> Torque ICE/1, Sum2/2
  Sum2/1 -> Gain/1  "Added, limited charge torque"
  Gain/1 -> Torque EM/1

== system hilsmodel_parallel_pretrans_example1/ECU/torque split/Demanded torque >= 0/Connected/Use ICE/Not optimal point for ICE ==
  Tdemand [Nm] : Inport
  Action Port : ActionPort  InitializeStates=reset  ActionType=then
  Constant : Constant  Value=dat.maxEngineTorque.value
  Gain : Gain  Gain=1/dat.finalgear.value
  Sum : Sum  Inputs=-+|
  Torque EM : Outport  OutputWhenDisabled=reset  InitialOutput=[0]
  Torque ICE : Outport  Port=2  OutputWhenDisabled=reset  InitialOutput=[0]
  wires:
  Constant/1 -> Torque ICE/1, Sum/1
  Gain/1 -> Torque EM/1
  Tdemand [Nm]/1 -> Sum/2
  Sum/1 -> Gain/1
